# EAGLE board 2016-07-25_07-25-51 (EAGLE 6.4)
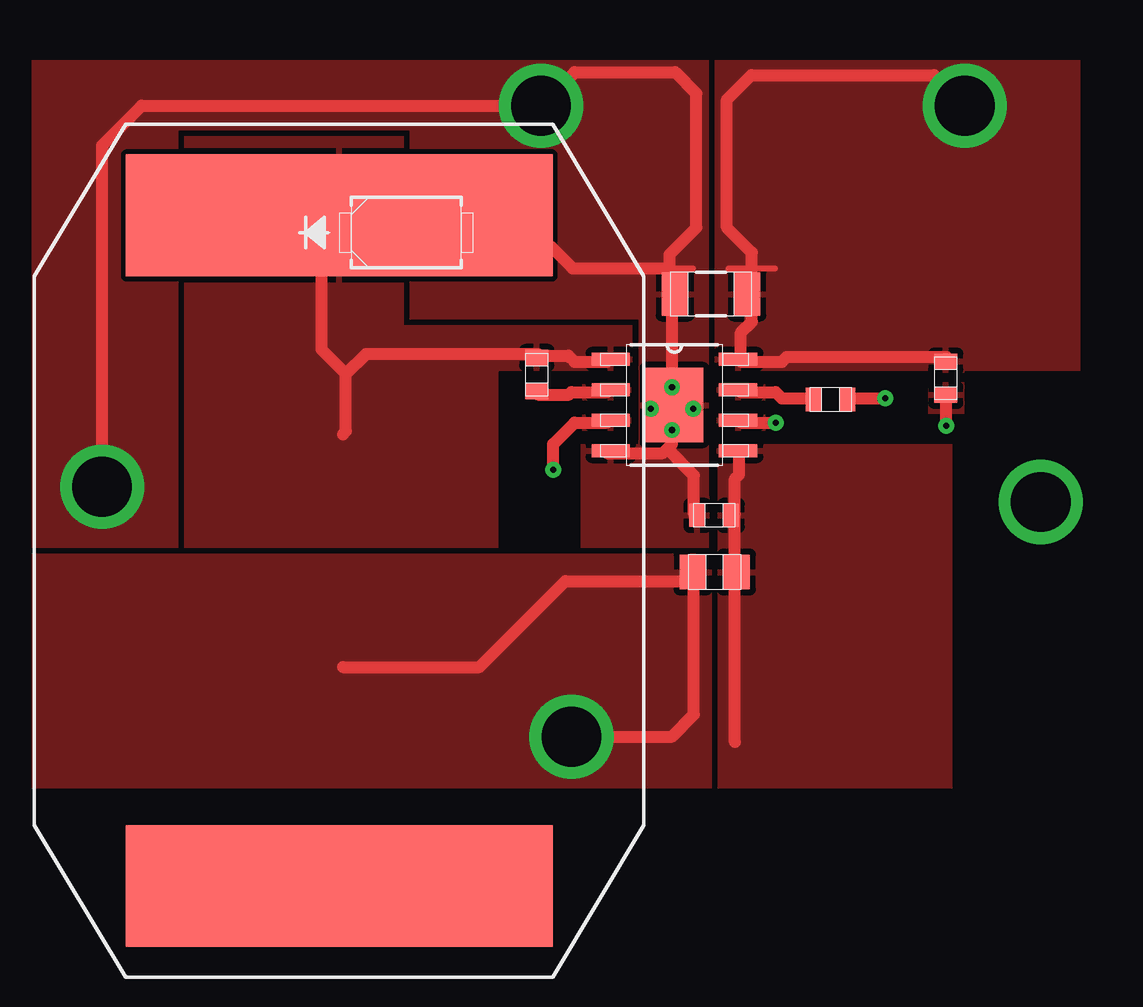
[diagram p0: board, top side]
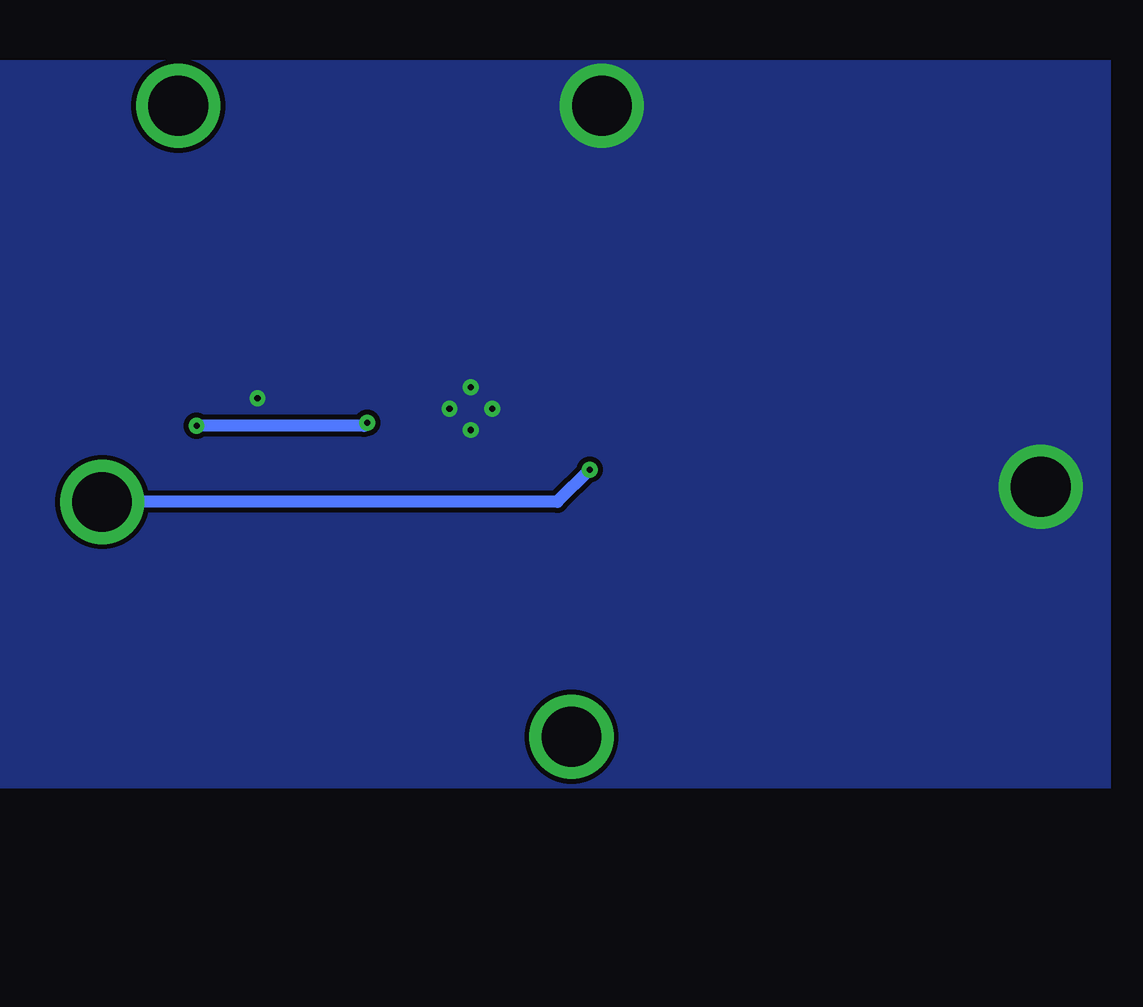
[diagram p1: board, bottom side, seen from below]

No outline drawn. Coordinates in mm, seen from the top.
Copper layers ((1*2)+(15*16)): TOP / INTERNAL1 / layer 15 / BOTTOM

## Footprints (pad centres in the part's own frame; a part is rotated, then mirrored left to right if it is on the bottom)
0603 = smd 0.66 x 0.965: 1 -0.699,0; 2 0.699,0
1206_190 = smd 1.118 x 1.803: 1 -1.499,0; 2 1.499,0
0805 = smd 1.118 x 1.448: 1 -0.902,0; 2 0.902,0
SMA = smd 2.184 x 1.626: 1 -1.854,0; 2 1.854,0
TP-1502 = drill 0.813 round: 1 0,0
PM2110 = smd 5.08 x 17.78: 1 -13.97,0; 2 13.97,0
MRA08B = smd 1.6 x 0.533: 1 -2.654,1.905; 2 -2.654,0.635; 3 -2.654,-0.635; 4 -2.654,-1.905; 5 2.654,-1.905; 6 2.654,-0.635; 7 2.654,0.635; 8 2.654,1.905 | smd 2.413 x 3.099: 9 0,0

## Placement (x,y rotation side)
Cb  [0603]  47.19,43.41 90 top
Cbyp  [0603]  59.44,42.37 0 top
Cin  [1206_190]  54.46,46.76 180 top
Cout  [0805]  54.61,35.18 0 top
D1  [SMA]  41.76,49.33 0 top
DIM  [TP-1502]  68.2,38.1 0 top
Gnd  [TP-1502]  47.32,54.58 0 top
Gnd1  [TP-1502]  29.06,38.73 0 top
L1  [PM2110]  38.96,36.07 270 top
Ron  [0603]  64.24,43.26 270 top
Rsns  [0603]  54.58,37.54 0 top
U1  [MRA08B]  52.93,42.14 0 top
Vin  [TP-1502]  65,54.58 0 top
Vout  [TP-1502]  48.59,28.27 0 top

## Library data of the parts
Cb = ultra-librarian; RefDes: Cb; Type: GRM188R71E103KA01D
Cbyp = ultra-librarian; RefDes: Cbyp; Type: GRM188R71E104KA01D
Cin = ultra-librarian; RefDes: Cin; Type: GRM31CR71H225KA88L
Cout = ultra-librarian; RefDes: Cout; Type: GRM21BR71H105KA12L
D1 = ultra-librarian; RefDes: D1; Type: MBRA160T3G
DIM = ultra-librarian; RefDes: DIM; Type: TP-1502
Gnd = ultra-librarian; RefDes: Gnd; Type: TP-1502
Gnd1 = ultra-librarian; RefDes: Gnd1; Type: TP-1502
L1 = ultra-librarian; RefDes: L1; Type: PM2110-102K-RC
Ron = ultra-librarian; RefDes: Ron; Type: CRCW06031M13FKEA
Rsns = ultra-librarian; RefDes: Rsns; Type: CRCW06032R55FKEA
U1 = ultra-librarian; RefDes: U1; Type: LM3402HVMR/NOPB
Vin = ultra-librarian; RefDes: Vin; Type: TP-1502
Vout = ultra-librarian; RefDes: Vout; Type: TP-1502

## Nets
0: Cbyp.2 Cin.2 D1.2 Gnd1.1 Gnd.1 Rsns.1 U1.4 U1.9
1: Cin.1 Ron.1 U1.8 Vin.1
2: Cout.2 Rsns.2 U1.5
3: Cb.2 D1.1 L1.1 U1.1
4: Ron.2 U1.6
5: Cout.1 L1.2 Vout.1
6: Cbyp.1 U1.7
7: Cb.1 U1.2
11: DIM.1 U1.3

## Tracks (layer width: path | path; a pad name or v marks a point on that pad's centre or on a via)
0  (via drill 0.25 pad 0.51, 2.49 pad 3.48)
  TOP 0.254: 51.77,47.83 53.7,47.83
  TOP 0.508: v29.08,38.73 29.08,52.96 30.73,54.61 v47.37,54.61 48.77,56.01 52.96,56.01 53.85,55.12 53.85,49.53 52.73,48.41 52.73,47.83 | 52.73,47.83 48.69,47.83 47.75,48.77 45.24,48.77 | 52.73,47.83 52.83,47.73 v52.83,42.88 52.83,41.99 v52.83,41.1 52.83,40.51 52.63,40.31 | 52.63,40.31 52.45,40.13 50.11,40.13 | 52.63,40.31 53.75,39.19 53.75,37.59 | 60.27,42.42 v61.72,42.42
  other vias: 51.94,41.99 53.72,41.99
  pour TOP (rank 6): 53.09,36.83 53.09,38.33 54.38,38.33 54.38,36.83
  pour TOP: 49.02,40.51 49.02,36.2 54.36,36.2 54.36,56.52 26.16,56.52 26.16,36.2 32.26,36.2 32.26,53.59 41.91,53.59 41.91,45.72 51.44,45.72 51.44,40.51
  pour BOTTOM: 26.16,26.16 26.16,56.52 74.3,56.52 74.3,26.16
1  (via drill 2.49 pad 3.48)
  TOP 0.254: 55.19,47.83 57.12,47.83
  TOP 0.508: v65.02,54.61 63.75,55.88 56.13,55.88 55.12,54.86 55.12,49.53 56.16,48.49 56.16,47.83 56.16,45.62 55.7,45.16 55.7,43.97 55.73,43.94 57.4,43.94 57.61,44.15 64.26,44.15
  pour TOP: 63.5,43.48 63.5,44.78 65,44.78 65,43.48
  pour TOP (rank 5): 54.61,43.56 54.61,56.52 69.85,56.52 69.85,43.56
2
  TOP 0.254: 55.44,34.21 55.44,35.36
  TOP 0.508: 55.45,28.09 55.45,34.8 55.45,37.59 | 55.7,40.13 55.63,40.06 55.63,39.24 55.45,39.06 55.45,37.59 | 55.45,37.59
  pour TOP (rank 4): 54.69,39.8 54.69,40.46 56.72,40.46 56.72,39.8
  pour TOP (rank 6): 54.74,26.16 64.52,26.16 64.52,40.51 54.74,40.51
3
  TOP 0.508: 39.24,43.43 38.23,44.45 38.23,48.67 38.3,48.77 | 39.12,40.92 39.24,41.05 39.24,43.43 | 39.24,43.43 40.08,44.27 47.24,44.27 47.32,44.2 48.51,44.2 48.77,43.94 50.11,43.94
  pour TOP (rank 5): 51.18,43.56 51.18,45.47 41.66,45.47 41.66,53.34 32.51,53.34 32.51,36.2 45.59,36.2 45.59,43.56
4  (via drill 0.25 pad 0.51)
  TOP 0.508: v64.26,41.27 64.26,42.44 | 55.7,41.4 v57.15,41.4
  BOTTOM 0.508: v64.26,41.27 57.28,41.27 v57.15,41.4
  pour TOP: 63.5,41.78 63.5,43.08 65,43.08 65,41.78
  pour TOP (rank 3): 54.69,41.07 54.69,41.73 56.72,41.73 56.72,41.07
5  (via drill 2.49 pad 3.48)
  TOP 0.254: 53.73,34.21 53.73,35.36
  TOP 0.508: v48.64,28.32 52.83,28.32 53.75,29.23 53.75,34.8 48.39,34.8 44.81,31.22 39.12,31.22
  pour TOP (rank 4): 54.48,35.94 26.16,35.94 26.16,26.16 54.48,26.16
6
  TOP 0.508: 58.57,42.42 57.4,42.42 57.15,42.67 55.7,42.67
  pour TOP (rank 3): 54.69,42.34 54.69,43 56.72,43 56.72,42.34
7
  TOP 0.508: 50.11,42.67 48.64,42.67 48.54,42.57 47.24,42.57
  pour TOP (rank 2): 49.1,42.34 49.1,43 51.13,43 51.13,42.34
11  (via drill 0.25 pad 0.51, 2.49 pad 3.48)
  TOP 0.508: 50.11,41.4 48.77,41.4 47.88,40.51 v47.88,39.45
  BOTTOM 0.508: DIM.1 49.23,38.1 v47.88,39.45
  other vias: 68.2,38.1
  pour TOP (rank 2): 49.1,41.07 49.1,41.73 51.13,41.73 51.13,41.07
